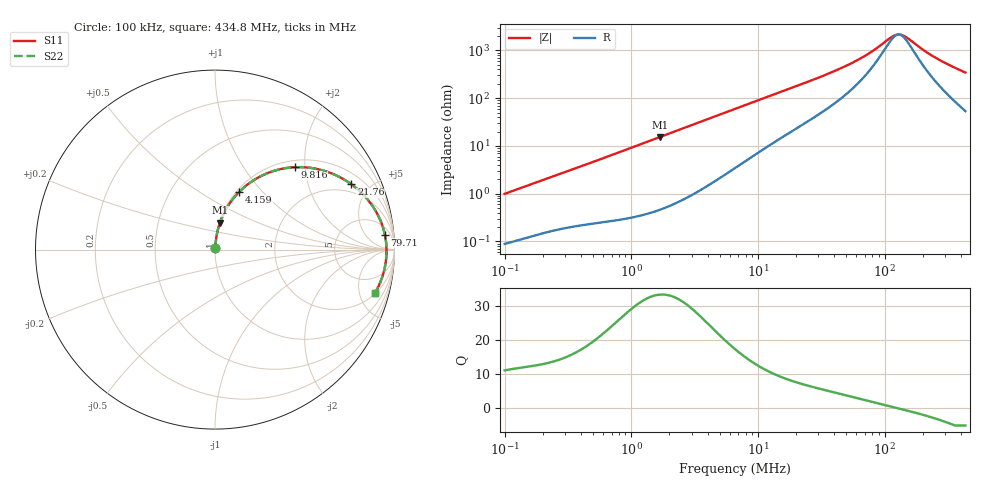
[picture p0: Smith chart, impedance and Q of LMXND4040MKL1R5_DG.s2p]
! LMXND4040MKL1R5_DG  S-PARAMETER MODEL  ( Standard Model )
! Model Generated by TAIYO YUDEN Corporation (http://www.ty-top.com)
! Version 1.0
! TAIYO YUDEN Control No. 20240226
! Copyright(c) 2024 TAIYO YUDEN CO.,LTD. All Rights Reserved.
! Product Description (link to TY-COMPAS)
! https://ds.yuden.co.jp/TYCOMPAS/or/detail?pn=LMXND4040MKL1R5NDG&u=M
! Products Name : Inductors
! Characteristics :
!  Inductance : 1.5 [uH] , SRF(min) : 90 [MHz] , DC Resistance(max) : 0.0612 [Ohm]
!  Rated Current : Saturation  2300 [mA] , Temp Rise  2000 [mA] (40 [degC])
!  Case Size : 4.0 x 4.0 / 0.157 x 0.157 [mm/inch] , Thickness : 1.2 / 0.047 [mm/inch]
!  (Conditions: Temperature = 25 [degC] , DC Bias Current = 0 [A])
! External Node Assignments :
!  1  o---GGG---o  2
! GND o---------o GND
! Frequency Range : 0.1MHz  -  434.768421MHz  [ 402 STEP ]
# MHz S RI R 50
! Freq[MHz].  S11 Real  S11 Imag  S21 Real  S21 Imag  S12 Real  S12 Imag  S22 Real  S22 Imag
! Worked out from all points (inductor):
!   401 points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, 100 kHz to 434.8 MHz, reference 50 ohm
!   read as one part in series: L = 1.56 uH near 104.3 kHz
!   highest Q = 33.3 at 1.69 MHz (marker M1), where L = 1.45 uH
!   self-resonance near 129.1 MHz
!   S11 on the Smith chart (normalised r, x): 100 kHz: 1.00, +0.02; 4.159 MHz: 1.03, +0.76; 9.816 MHz: 1.14, +1.76; 21.76 MHz: 1.53, +3.83; 79.71 MHz: 10, +17; 434.8 MHz: 2.07, -6.83
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0.1  0.000984 0.00987  0.999 -0.00987  0.999 -0.00987  0.000984 0.00987
0.406826  0.0036 0.0377  0.9964 -0.0377  0.9964 -0.0377  0.0036 0.0377
0.882972  0.0094 0.08  0.9906 -0.08  0.9906 -0.08  0.0094 0.08
1.65507  0.0266 0.1465  0.9734 -0.1465  0.9734 -0.1465  0.0266 0.1465
1.690099  0.0276 0.1494  0.9724 -0.1494  0.9724 -0.1494  0.0276 0.1494
2.793879  0.0678 0.2354  0.9322 -0.2354  0.9322 -0.2354  0.0678 0.2354
4.159344  0.1353 0.3221  0.8647 -0.3221  0.8647 -0.3221  0.1353 0.3221
6.733248  0.2827 0.422  0.7173 -0.422  0.7173 -0.422  0.2827 0.422
9.816264  0.4435 0.4591  0.5565 -0.4591  0.5565 -0.4591  0.4435 0.4591
14.01433  0.6012 0.4411  0.3988 -0.4411  0.3988 -0.4411  0.6012 0.4411
21.75609  0.7602 0.3637  0.2398 -0.3637  0.2398 -0.3637  0.7602 0.3637
26.82484  0.8161 0.3164  0.1839 -0.3164  0.1839 -0.3164  0.8161 0.3164
50.28131  0.9167 0.1739  0.0833 -0.1739  0.0833 -0.1739  0.9167 0.1739
64.64788  0.9361 0.123  0.0639 -0.123  0.0639 -0.123  0.9361 0.123
79.70962  0.9464 0.0837  0.0536 -0.0837  0.0536 -0.0837  0.9464 0.0837
109.1303  0.9545 0.0285  0.0455 -0.0285  0.0455 -0.0285  0.9545 0.0285
123.7426  0.9556 0.00716  0.0444 -0.00716  0.0444 -0.00716  0.9556 0.00716
131.7669  0.9559 -0.0035  0.0441 0.0035  0.0441 0.0035  0.9559 -0.0035
140.3115  0.9558 -0.0142  0.0442 0.0142  0.0442 0.0142  0.9558 -0.0142
246.9878  0.9423 -0.1167  0.0577 0.1167  0.0577 0.1167  0.9423 -0.1167
331.1423  0.9223 -0.1787  0.0777 0.1787  0.0777 0.1787  0.9223 -0.1787
434.7684  0.8903 -0.2436  0.1097 0.2436  0.1097 0.2436  0.8903 -0.2436
